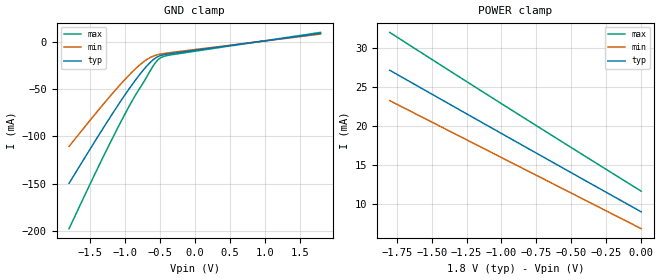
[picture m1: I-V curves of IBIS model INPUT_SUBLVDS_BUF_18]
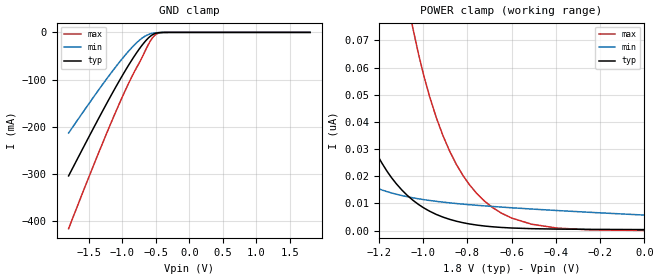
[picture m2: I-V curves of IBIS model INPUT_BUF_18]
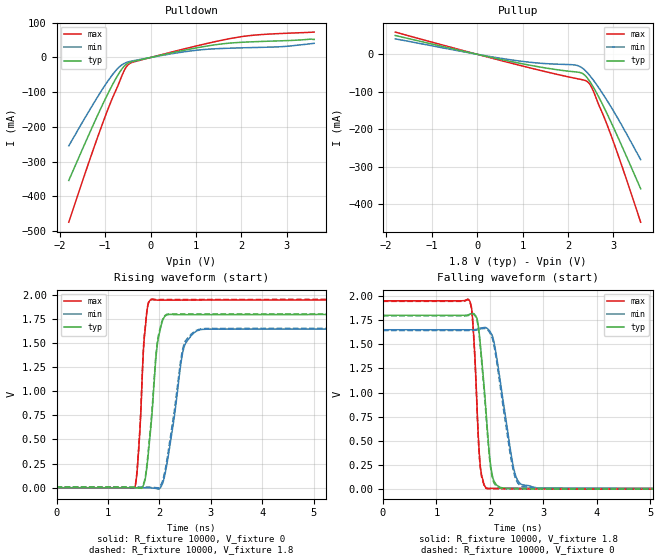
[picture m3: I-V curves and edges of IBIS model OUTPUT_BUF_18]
| TEXAS INSTRUMENTS INCORPORATED
| Digital Light Processing Group
| IBIS Model of D1111HX2SV
| P55_GEN2_AUTO
| This device can be powered at the following Vccs:
|  1.8 volt Vcc
| This file provides unique models under the [Model Selector] for each Vcc.
| For operation at a specific Vcc, select the appropriate model after each
| [Model Selector] keyword.
[IBIS Ver]   3.2
[Comment char]  |_char
[File Name]   d1111hx2sv.ibs
[File Rev]   1.0 | f_die
[Date]   February 16, 2016
[Source]   Data created from TI-SPICE simulations at TI-DLP.
[Notes]   The following is an IBIS list for the P55_GEN2_AUTO.
##notes##|
[Disclaimer] Property of Texas Instruments Incorporated.  Unauthorized
   reproduction and/or distribution is strictly prohibited.
   This product is protected under copyright law.
   Created  2014, (C) Copyright  2014, Texas Instruments
   Incorporated, All Rights Reserved
   UNLESS THERE IS A SIGNED, WRITTEN AGREEMENT TO THE
   CONTRARY, TEXAS INSTRUMENTS (TI) IS PROVIDING THE IBIS
   MODELS  AND WITHOUT ANY WARRANTY, EXPRESSED OR
   IMPLIED.  TI assumes no liability for:
   1) the accuracy of the IBIS models provided to your
   company;
   2) the proper functioning of these IBIS Models in your
   design or for any resulting applications; or
   3) infringement of patents, copyrights or intellectual
   property rights resulting from your use of these IBIS
   models.
   TI provides IBIS Models as a service to our customers.
   You and your company shall not distribute, sell or give
   these models to anyone else without prior written
   permission from TI.
   TI reserves the right to make changes to our products or
   to discontinue any semiconductor product or service
   without notice, and advises our customers to obtain the
   latest version of relevant information to verify, before
   placing orders, that the information being relied on is
   current.
   Please be aware that your receipt and use of the IBIS
   information provided shall serve as acceptance of these
   terms and conditions.  If you do not accept these terms,
   you should return or destroy the IBIS models and any
   other accompanying information immediately.
| Component P55_GEN2_AUTO_PW 149-pin PGA
[Component]   P55_GEN2_AUTO_PW
[Manufacturer]   Texas Instruments, Inc.
[Package]
|   typ   min   max
R_pkg   7.570E-01   3.164E-01   1.297E+00
L_pkg   3.607E-09   1.961E-09   5.740E-09
C_pkg   1.200E-12   7.085E-13   1.835E-12
[Pin]   signal_name   model_name   R_pin   L_pin   C_pin
T17   MBRST<0>   NC
T18   MBRST<1>   NC
R18   MBRST<2>   NC
R19   MBRST<3>   NC
R17   MBRST<4>   NC
P18   MBRST<5>   NC
R16   MBRST<6>   NC
P19   MBRST<7>   NC
T12   TP0   NC
M19   TP1   NC
R12   TP2   NC
K20   D_BP<0>   INPUT_SUB_LVDS_BUF   1.066E+00   5.000E-09   3.100E-12
K19   D_BN<0>   INPUT_SUB_LVDS_BUF   1.131E+00   5.100E-09   3.500E-12
J20   D_BP<1>   INPUT_SUB_LVDS_BUF   9.640E-01   4.600E-09   3.200E-12
J19   D_BN<1>   INPUT_SUB_LVDS_BUF   1.049E+00   4.800E-09   3.500E-12
H20   D_BP<2>   INPUT_SUB_LVDS_BUF   9.530E-01   4.600E-09   3.200E-12
H19   D_BN<2>   INPUT_SUB_LVDS_BUF   9.890E-01   4.700E-09   3.100E-12
G20   D_BP<3>   INPUT_SUB_LVDS_BUF   9.680E-01   4.500E-09   3.100E-12
G19   D_BN<3>   INPUT_SUB_LVDS_BUF   1.029E+00   4.800E-09   2.900E-12
F20   DCLK_BP   INPUT_SUB_LVDS_BUF   1.041E+00   4.900E-09   3.000E-12
F19   DCLK_BN   INPUT_SUB_LVDS_BUF   1.076E+00   5.000E-09   3.000E-12
E20   D_BP<4>   INPUT_SUB_LVDS_BUF   1.367E+00   5.800E-09   3.300E-12
E19   D_BN<4>   INPUT_SUB_LVDS_BUF   1.457E+00   6.100E-09   3.600E-12
D20   D_BP<5>   INPUT_SUB_LVDS_BUF   1.547E+00   6.500E-09   3.600E-12
D19   D_BN<5>   INPUT_SUB_LVDS_BUF   1.608E+00   6.800E-09   3.500E-12
C20   D_BP<6>   INPUT_SUB_LVDS_BUF   1.532E+00   6.500E-09   3.700E-12
C19   D_BN<6>   INPUT_SUB_LVDS_BUF   1.593E+00   6.700E-09   3.600E-12
B20   D_BP<7>   INPUT_SUB_LVDS_BUF   1.582E+00   6.800E-09   3.600E-12
B19   D_BN<7>   INPUT_SUB_LVDS_BUF   1.620E+00   6.800E-09   4.200E-12
C2   D_AN<7>   INPUT_SUB_LVDS_BUF   1.489E+00   6.300E-09   3.600E-12
C1   D_AP<7>   INPUT_SUB_LVDS_BUF   1.449E+00   6.100E-09   3.800E-12
D2   D_AN<6>   INPUT_SUB_LVDS_BUF   1.401E+00   6.000E-09   3.600E-12
D1   D_AP<6>   INPUT_SUB_LVDS_BUF   1.338E+00   5.800E-09   3.500E-12
E2   D_AN<5>   INPUT_SUB_LVDS_BUF   1.407E+00   6.000E-09   3.700E-12
E1   D_AP<5>   INPUT_SUB_LVDS_BUF   1.347E+00   5.800E-09   3.600E-12
F2   D_AN<4>   INPUT_SUB_LVDS_BUF   1.209E+00   5.300E-09   3.400E-12
F1   D_AP<4>   INPUT_SUB_LVDS_BUF   1.121E+00   4.900E-09   2.800E-12
G2   DCLK_AN   INPUT_SUB_LVDS_BUF   9.650E-01   4.400E-09   2.900E-12
G1   DCLK_AP   INPUT_SUB_LVDS_BUF   9.290E-01   4.700E-09   3.300E-12
H2   D_AN<3>   INPUT_SUB_LVDS_BUF   1.030E+00   4.700E-09   2.600E-12
H1   D_AP<3>   INPUT_SUB_LVDS_BUF   9.680E-01   4.600E-09   2.800E-12
J2   D_AN<2>   INPUT_SUB_LVDS_BUF   1.086E+00   4.900E-09   3.000E-12
J1   D_AP<2>   INPUT_SUB_LVDS_BUF   1.047E+00   4.800E-09   3.100E-12
K2   D_AN<1>   INPUT_SUB_LVDS_BUF   1.127E+00   5.200E-09   3.300E-12
K1   D_AP<1>   INPUT_SUB_LVDS_BUF   1.041E+00   4.800E-09   2.800E-12
L2   D_AN<0>   INPUT_SUB_LVDS_BUF   1.277E+00   5.800E-09   3.800E-12
L1   D_AP<0>   INPUT_SUB_LVDS_BUF   1.211E+00   5.400E-09   3.200E-12
P1   TEMP_N   NC
N1   TEMP_P   NC
T10   DMD_DEN_ARSTZ INPUT_BUF   1.974E+00   1.000E-08   4.800E-12
T6   LS_RDATA_B   OUTPUT_BUF   1.406E+00   7.700E-09   4.200E-12
T5   LS_RDATA_A   OUTPUT_BUF   1.324E+00   7.200E-09   3.700E-12
R2   LS_WDATA_N   INPUT_SUB_LVDS_BUF   1.818E+00   7.500E-09   4.100E-12
T2   LS_WDATA_P   INPUT_SUB_LVDS_BUF   1.793E+00   7.600E-09   3.900E-12
R3   LS_CLK_N   INPUT_SUB_LVDS_BUF   1.885E+00   7.700E-09   4.400E-12
T3   LS_CLK_P   INPUT_SUB_LVDS_BUF   1.870E+00   7.700E-09   4.500E-12
A3   VSS   GND
A4   VSS   GND
A5   VOFFSET   POWER
A6   VDD   POWER
A7   VSS   GND
A8   VCCH   POWER
A9   VCCH   POWER
A10   VCCH   POWER
A11   VSSH   POWER
A12   VSSH   POWER
A13   VSSH   POWER
A14   NO_CONNECT   NC
A15   VSS   GND
A16   VOFFSET   POWER
A17   VSS   GND
A18   VDD   POWER
A19   VSS   GND
A20   VSS   GND
B2   VSS   GND
B3   VDDI   POWER
B4   VSS   GND
B5   VOFFSET   POWER
B6   NO_CONNECT   NC
B7   NO_CONNECT   NC
B8   VCCH   POWER
B9   VCCH   POWER
B10   VCCH   POWER
B11   VSSH   POWER
B12   VSSH   POWER
B13   VSSH   POWER
B14   NO_CONNECT   NC
B15   VSS   GND
B16   VOFFSET   POWER
B17   VSS   GND
B18   VDDI   POWER
C3   VDD   POWER
C18   VSS   GND
D3   VSS   GND
D18   VDD   POWER
E3   VDD   POWER
E18   VDDI   POWER
F3   VDDI   POWER
F18   VSS   GND
G3   VSS   GND
G18   VDD   POWER
H3   VDD   POWER
H18   VDDI   POWER
J3   VDDI   POWER
J18   VSS   GND
K3   VSS   GND
K18   VDD   POWER
L3   VDD   POWER
L18   VDDI   POWER
L19   VSS   GND
L20   VSS   GND
M1   VSS   GND
M2   VSS   GND
M3   VDDI   POWER
M18   NO_CONNECT   NC
M20   VDD   POWER
N2   VDD   POWER
N3   NO_CONNECT   NC
N18   NO_CONNECT   NC
N19   VSS   GND
N20   VSS   GND
P2   VSS   GND
P3   VSS   GND
P20   VSS   GND
R1   VDDI   POWER
R4   VDD   POWER
R5   VSS   GND
R6   VSS   GND
R7   VSS   GND
R8   VSS   GND
R9   VSS   GND
R10   VDD   POWER
R11   VDD   POWER
R13   VSS   GND
R14   VSS   GND
R15   VSS   GND
R20   VDD   POWER
T1   VSS   GND
T4   VDDI   POWER
T7   VBIAS   POWER
T8   VRESET   POWER
T9   VOFFSET   POWER
T11   NO_CONNECT   NC
T13   VOFFSET   POWER
T14   VRESET   POWER
T15   VBIAS   POWER
T16   VSS   GND
T19   VSS   GND
T20   VSS   GND
| NOTE:  The [Diff Pin] section may get flagged by early versions of the
|   ibischk program
[Diff Pin]  inv_pin   vdiff   tdelay_typ
L1   L2   200mv   NA
K1   K2   200mv   NA
J1   J2   200mv   NA
H1   H2   200mv   NA
F1   F2   200mv   NA
E1   E2   200mv   NA
D1   D2   200mv   NA
C1   C2   200mv   NA
G1   G2   200mv   NA
K20   K19   200mv   NA
J20   J19   200mv   NA
H20   H19   200mv   NA
G20   G19   200mv   NA
E20   E19   200mv   NA
D20   D19   200mv   NA
C20   C19   200mv   NA
B20   B19   200mv   NA
F20   F19   200mv   NA
T2   R2   200mv   NA
T3   R3   200mv   NA   |
| Model INPUT_SUB_LVDS_BUF
[Model Selector]   INPUT_SUB_LVDS_BUF
INPUT_SUBLVDS_BUF_18   1.8 volt Vcc
| Model INPUT_BUF
[Model Selector]   INPUT_BUF
INPUT_BUF_18   1.8 volt Vcc
| Model OUTPUT_BUF
[Model Selector]   OUTPUT_BUF
OUTPUT_BUF_18   1.8 volt Vcc
| Models and submodels in the file (3): INPUT_SUBLVDS_BUF_18 (Input), INPUT_BUF_18 (Input), OUTPUT_BUF_18 (Output)
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[Model]   INPUT_SUBLVDS_BUF_18
Model_type  Input
Vinl=0.80
Vinh=1.00
| variable   typ   min   max
C_comp   0.69pF   0.66pF   0.72pF
[Temperature Range]   25   85   -40
[Voltage range]   1.8   1.65   1.95
[GND Clamp]
| INPUT_SUBLVDS_BUF_18
|   Voltage   I(typ)   I(min)   I(max)
-1.8V     -149.7mA   -110.7mA   -197.8mA
-1.29V    -88.84mA   -64.29mA   -118.6mA
-1.095V   -66.55mA   -47.56mA   -89.83mA
-930mV    -48.67mA   -34.42mA   -66.87mA
-790mV    -34.7mA    -24.56mA   -49.3mA
-680mV    -25.03mA   -18.39mA   -35.98mA
-580mV    -18.08mA   -14.73mA   -23.73mA
-510mV    -15.09mA   -13.26mA   -17.94mA
-450mV    -13.75mA   -12.43mA   -15.53mA
-355mV    -12.57mA   -11.45mA   -13.96mA
1.8V      8.993mA    8.203mA    9.976mA
[POWER Clamp]
| INPUT_SUBLVDS_BUF_18
|   Voltage   I(typ)   I(min)   I(max)
-1.8V     27.16mA    23.26mA    32.02mA
-1.37V    22.79mA    19.34mA    27.08mA
-920mV    18.24mA    15.23mA    21.97mA
-16.28fV  8.993mA    6.835mA    11.65mA
[Model]   INPUT_BUF_18
Model_type  Input
Vinl=0.54
Vinh=1.26
| variable   typ   min   max
C_comp   0.51pF   0.44pF   0.58pF
[Temperature Range]   25   85   -40
[Voltage range]   1.8   1.65   1.95
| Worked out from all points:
|   GND clamp passes 1 mA (typ) near -0.47 V on its own axis
[GND Clamp]
| INPUT_BUF_18
|   Voltage   I(typ)   I(min)   I(max)
-1.8V     -304mA     -213.1mA   -415.8mA
-1.52V    -227.4mA   -155.6mA   -314.4mA
-1.29V    -165.7mA   -109.6mA   -233.4mA
-1.095V   -115.3mA   -72.59mA   -167.6mA
-930mV    -75.06mA   -43.75mA   -115.2mA
-790mV    -43.93mA   -22.51mA   -75.55mA
-680mV    -22.72mA   -9.755mA   -45.56mA
-580mV    -7.998mA   -2.996mA   -17.96mA
-510mV    -2.379mA   -972.8uA   -5.564mA
-450mV    -592.5uA   -304.6uA   -1.296mA
-355mV    -35.15uA   -32.8uA    -61.22uA
1.8V      384pA      6.33nA     42.47pA
[POWER Clamp]
| INPUT_BUF_18
|   Voltage   I(typ)   I(min)   I(max)
-1.8V     438.6nA    109.4nA    1.836uA
-1.7V     293.4nA    73.99nA    1.296uA
-1.565V   164.4nA    44.27nA    784.1nA
-1.4V     75.97nA    25.31nA    401.7nA
-1.255V   36.21nA    17.25nA    210.8nA
-1.155V   20.97nA    14.17nA    130.5nA
-1.045V   11.14nA    12.07nA    74.21nA
-970mV    7.14nA     11.1nA     49.29nA
-880mV    4.163nA    10.23nA    29.33nA
-685mV    1.408nA    8.888nA    8.453nA
-395mV    567.5pA    7.406nA    949.3pA
-16.28fV  384pA      5.724nA    60.79pA
[Model]   OUTPUT_BUF_18
Model_type  Output
Vref =   0
Rref =   10000
Cref =   10p
Vmeas =   1.2
| variable   typ   min   max
C_comp   0.65pF   0.45pF   1.15pF
| C_pullup   0.66pF   0.45pF   1.15pF
| C_pulldown   0.63pF   0.50pF   1.03pF
[Temperature Range]   25   85   -40
[Voltage range]   1.8   1.65   1.95
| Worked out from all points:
|   slope of the pulldown table from 0 to 0.27 V, typ, clamps not added: 34.3 ohm
|   slope of the pullup table from 0 to 0.27 V, typ, clamps not added: 37.6 ohm
|   rising waveform, R_fixture 10000, V_fixture 0: 20-80 % time 164ps typ, 253ps min, 111ps max; typ from 0 V to 1.79 V
|   falling waveform, R_fixture 10000, V_fixture 1.8: 20-80 % time 159ps typ, 266ps min, 98.4ps max; typ from 1.8 V to 0.006 V
|   rising waveform, R_fixture 10000, V_fixture 1.8: 20-80 % time 164ps typ, 256ps min, 110ps max; typ from 0.006 V to 1.8 V
|   falling waveform, R_fixture 10000, V_fixture 0: 20-80 % time 159ps typ, 263ps min, 98.5ps max; typ from 1.79 V to 0 V
[Pulldown]
| OUTPUT_BUF_18
|   Voltage   I(typ)   I(min)   I(max)
-1.8V     -354.2mA   -254.4mA   -474.4mA
-1.265V   -195mA     -134.5mA   -266.6mA
-895mV    -92.67mA   -59.47mA   -134.6mA
-755mV    -58.61mA   -36.11mA   -91.94mA
-645mV    -35.65mA   -22.4mA    -56.96mA
-555mV    -21.67mA   -15.53mA   -31.37mA
-480mV    -15.3mA    -12.24mA   -19.11mA
-345mV    -10.18mA   -8.457mA   -11.8mA
875mV     24.33mA    18.74mA    29.04mA
1.865V    42.67mA    27.28mA    57.21mA
2.905V    48.22mA    31.33mA    69.32mA
3.6V      52.02mA    40.86mA    73.18mA
[Pullup]
| OUTPUT_BUF_18
|   Voltage   I(typ)   I(min)   I(max)
-1.8V     49.99mA    41.08mA    59.07mA
730mV     -18.9mA    -14.55mA   -23.06mA
1.36V     -33.47mA   -23.55mA   -42.08mA
2.165V    -46.93mA   -28.87mA   -64.13mA
2.32V     -51.32mA   -37.02mA   -67.96mA
2.435V    -64.68mA   -50.22mA   -73.6mA
2.49V     -74.19mA   -58.09mA   -81.45mA
2.545V    -84.87mA   -66.63mA   -94.28mA
2.7V      -119.1mA   -93.19mA   -140.9mA
2.895V    -167.2mA   -129.8mA   -198.5mA
3.195V    -246.7mA   -191.5mA   -300.4mA
3.6V      -358.2mA   -280.8mA   -447.3mA
[Ramp]
| OUTPUT_BUF_18
| variable   typ   min   max
dV/dt_r   1.08/1.67E-10   0.99/2.58E-10   1.17/1.11E-10
dV/dt_f   1.09/1.62E-10   1.00/2.72E-10   1.18/1.01E-10
R_load = 10000
[Rising Waveform]
| OUTPUT_BUF_18
R_fixture =   10000
C_fixture =   0
L_fixture =   0
V_fixture =   0
V_fixture_min = 0
V_fixture_max = 0
|   Time   V(typ)   V(min)   V(max)
0s        2.935nV    32.33nV    304.2pV
1.525ns   12.81uV    20.21uV    4.084mV
1.615ns   -3.833mV   105uV      533.5mV
1.71ns    58.13mV    123.1uV    1.568V
1.855ns   750.8mV    -2.782mV   1.947V
1.955ns   1.458V     -9.919mV   1.942V
2.08ns    1.753V     73.73mV    1.941V
2.47ns    1.791V     1.436V     1.942V
2.825ns   1.792V     1.638V     1.943V
24.99ns   1.793V     1.642V     1.944V
[Falling Waveform]
| OUTPUT_BUF_18
R_fixture =   10000
C_fixture =   0
L_fixture =   0
V_fixture =   1.8
V_fixture_min = 1.65
V_fixture_max = 1.95
|   Time   V(typ)   V(min)   V(max)
0s        1.8V       1.65V      1.95V
1.62ns    1.81V      1.65V      1.949V
1.69ns    1.819V     1.651V     1.653V
1.76ns    1.764V     1.656V     844.3mV
1.82ns    1.507V     1.667V     244.5mV
1.955ns   601.1mV    1.662V     9.6mV
2.08ns    79.45mV    1.512V     9.328mV
2.475ns   9.39mV     152mV      8.293mV
2.885ns   8.404mV    13.17mV    7.567mV
24.99ns   6.04mV     6.675mV    5.66mV
[Rising Waveform]
| OUTPUT_BUF_18
R_fixture =   10000
C_fixture =   0
L_fixture =   0
V_fixture =   1.8
V_fixture_min = 1.65
V_fixture_max = 1.95
|   Time   V(typ)   V(min)   V(max)
0s        6.039mV    6.675mV    5.66mV
1.525ns   6.058mV    6.695mV    10.55mV
1.61ns    2.738mV    6.771mV    514.5mV
1.71ns    72.65mV    6.795mV    1.588V
1.855ns   789.8mV    4.171mV    1.952V
1.955ns   1.486V     187.2uV    1.948V
2.08ns    1.761V     104.7mV    1.948V
2.465ns   1.798V     1.459V     1.948V
2.825ns   1.798V     1.646V     1.949V
24.99ns   1.8V       1.65V      1.95V
[Falling Waveform]
| OUTPUT_BUF_18
R_fixture =   10000
C_fixture =   0
L_fixture =   0
V_fixture =   0
V_fixture_min = 0
V_fixture_max = 0
|   Time   V(typ)   V(min)   V(max)
0s        1.793V     1.642V     1.944V
1.62ns    1.803V     1.642V     1.942V
1.69ns    1.811V     1.643V     1.63V
1.76ns    1.748V     1.648V     814.7mV
1.815ns   1.504V     1.657V     253.2mV
1.955ns   560.3mV    1.649V     4.112mV
2.075ns   66.14mV    1.49V      3.651mV
2.465ns   3.348mV    135.5mV    2.653mV
2.86ns    2.404mV    7.718mV    1.943mV
24.99ns   6.498nV    37.43nV    3.212nV
